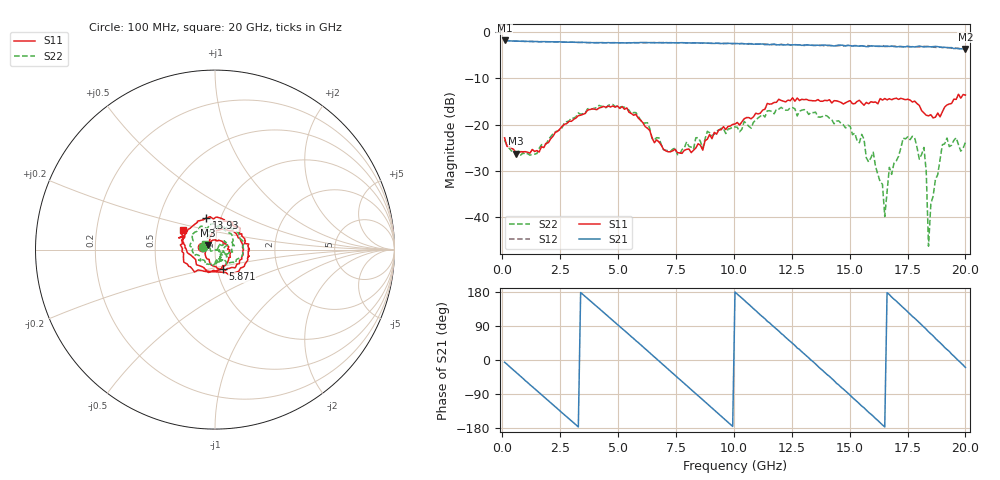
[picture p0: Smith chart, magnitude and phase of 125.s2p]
!Agilent Technologies,N5230C,MY49001569,A.09.33.09
!Agilent N5230C: A.09.33.09
!Date: Friday, July 24, 2015 10:45:00
!Correction: S11(Full 2 Port(1,2))
!S21(Full 2 Port(1,2))
!S12(Full 2 Port(1,2))
!S22(Full 2 Port(1,2))
!S2P File: Measurements: S11, S21, S12, S22:
# Hz S  dB  R 50
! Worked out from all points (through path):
!   201 points, 100 MHz to 20 GHz, reference 50 ohm
!   highest |S21| = -1.85 dB at 100 MHz (marker M1); lowest = -3.7 dB at 20 GHz (marker M2)
!   group delay of S21, straight-line fit = 152 ps
!   lowest |S11| = -26.3 dB at 597.5 MHz (marker M3), VSWR 1.10, Z = 46 + j2.43 ohm
!   |S11| at or under -10 dB: start of sweep to end of sweep
!   |S22| runs from -46.2 to -15.7 dB; largest |S21 - S12| = 0.02
!   S11 on the Smith chart (normalised r, x): 100 MHz: 0.87, +0.03; 5.871 GHz: 1.06, -0.24; 13.93 GHz: 0.86, +0.31; 20 GHz: 0.68, +0.16
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1e8  -22.85 167.3  -1.85 -5.9  -1.84 -5.9  -23.39 169.2
5.975e8  -26.28 147.2  -1.98 -32.8  -1.99 -32.8  -25.98 149.4
1.891e9  -24.03 118.5  -2.10 -102.2  -2.11 -102.4  -24.21 129.7
3.483e9  -17.78 55.0  -2.24 172.8  -2.27 172.6  -17.63 72.7
4.7765e9  -15.97 -9.8  -2.33 104.0  -2.33 104.1  -15.66 11.6
5.871e9  -18.58 -68.5  -2.33 46.0  -2.33 45.3  -18.17 -34.7
6.7665e9  -23.76 -141.8  -2.32 -2.7  -2.30 -2.6  -22.87 -54.0
8.3585e9  -25.02 69.5  -2.36 -89.0  -2.41 -88.9  -22.82 -78.7
1.005e10  -19.86 -52.6  -2.52 179.2  -2.51 179.3  -20.48 -125.5
1.17415e10  -15.21 -147.6  -2.64 86.8  -2.70 86.4  -17.66 159.2
1.3433e10  -14.86 130.1  -2.92 -4.9  -2.88 -4.8  -17.42 71.4
1.39305e10  -14.75 105.0  -2.83 -33.0  -3.06 -33.2  -17.97 44.9
1.49255e10  -15.03 62.8  -2.88 -87.8  -2.93 -88.0  -20.12 -7.8
1.602e10  -15.20 17.1  -3.02 -148.2  -3.13 -149.0  -25.95 -35.0
1.65175e10  -14.37 0.4  -3.08 -176.6  -3.16 -177.8  -39.82 -35.5
1.67165e10  -14.40 -2.5  -3.14 172.7  -3.15 171.8  -29.21 47.0
1.8209e10  -17.46 -70.3  -3.25 87.0  -3.12 86.6  -24.92 -18.3
1.83085e10  -17.98 -81.5  -3.19 81.2  -3.12 81.0  -30.10 -14.3
1.8408e10  -18.10 -98.4  -3.18 74.5  -3.14 74.7  -46.22 -11.7
1.85075e10  -17.86 -110.2  -3.21 69.1  -3.22 69.9  -37.12 -138.6
1.9005e10  -17.24 -166.8  -3.33 39.7  -3.38 39.0  -24.33 158.0
2e10  -13.62 148.2  -3.67 -19.6  -3.91 -19.5  -23.85 152.8
